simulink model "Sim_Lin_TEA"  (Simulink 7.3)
settings: Solver=ode113  StartTime=0.0  StopTime=100000  RelTol=1e-3
InitFcn:
  | start3
StopFcn:
  | Pl3
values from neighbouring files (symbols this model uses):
  Kpqr = lqr(sys,Q0,R0)    [des.m]
  r2d = 180/pi    (= 57.2957795131)    [start.m]    (also in start1.m; start2.m; start3.m)
  wo = 0.0011    [start.m]    (also in start1.m; start2.m; start3.m)
undefined symbols (not defined in the file or in its folder): Linear2_LVLH

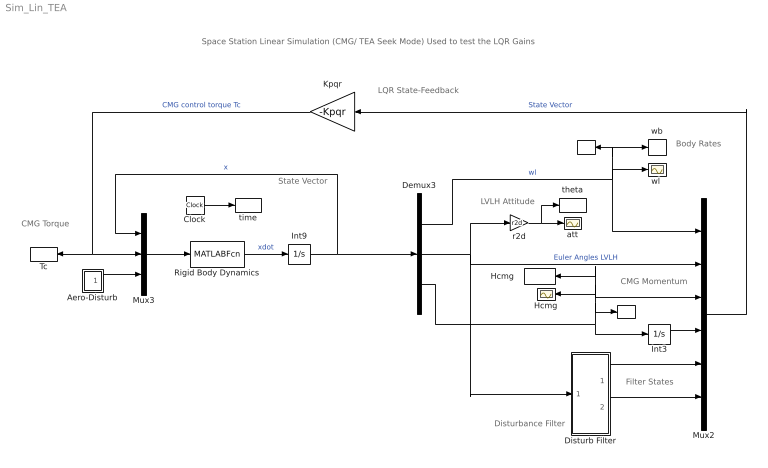
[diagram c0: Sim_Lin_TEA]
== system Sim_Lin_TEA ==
  note: Space Station Linear Simulation (CMG/ TEA Seek Mode) Used to test the LQR Gains
  note: State Vector
  note: LQR State-Feedback
  note: Body Rates
  note: CMG Momentum
  note: LVLH Attitude
  note: Filter States
  note: Disturbance Filter
  note: CMG Torque
  " " : ToWorkspace  VariableName=wl  SampleTime=-1  SaveFormat=Array
  "  " : ToWorkspace  VariableName=Hsys  SampleTime=-1  SaveFormat=Array
  Aero-Disturb : Subsystem
  Clock : Clock
  Demux3 : Demux  Outputs=[3,3,3]
  Disturb Filter : Subsystem
  Hcmg : Scope
  "Hcmg  " : ToWorkspace  VariableName=Hcmg  SampleTime=-1  SaveFormat=Array
  Int3 : Integrator
  Int9 : Integrator
  Kpqr : Gain  Gain=-Kpqr  Multiplication=Matrix(K*u)  ParameterDataType=sfix(16)  ParameterScaling=2^0  OutDataType=sfix(16)  OutScaling=2^0
  Mux2 : Mux  Inputs=[3, 3, 3, 3, 1, 1]
  Mux3 : Mux  Inputs=[9, 3, 3]
  Rigid Body Dynamics : MATLABFcn  MATLABFcn=Linear2_LVLH( u(1:9), u(10:12), u(13:15) )  OutputDimensions=9
  Tc : ToWorkspace  VariableName=Tcmg  SampleTime=-1  SaveFormat=Array
  att : Scope
  r2d : Gain  Gain=r2d  ParameterDataType=sfix(16)  ParameterScaling=2^0  OutDataType=sfix(16)  OutScaling=2^0
  theta : ToWorkspace  VariableName=theta  SampleTime=-1  SaveFormat=Array
  time : ToWorkspace  VariableName=time  SampleTime=-1  SaveFormat=Array
  wb : ToWorkspace  VariableName=wb  SampleTime=-1  SaveFormat=Array
  "wl " : Scope
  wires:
  Int3/1 -> Mux2/4
  Demux3/3 -> Int3/1, Hcmg/1, "Hcmg  "/1, Mux2/3, "  "/1
  Demux3/2 -> r2d/1, Mux2/2, Disturb Filter/1(the)  "Euler Angles LVLH"
  Kpqr/1 -> Tc/1, Mux3/2  "CMG control torque Tc"
  Int9/1 -> Demux3/1, Mux3/1  "x"
  Rigid Body Dynamics/1 -> Int9/1  "xdot"
  Demux3/1 -> "wl "/1, Mux2/1, wb/1, " "/1  "wl"
  Aero-Disturb/1(Td) -> Mux3/3
  r2d/1 -> att/1, theta/1
  Mux2/1 -> Kpqr/1  "State Vector"
  Clock/1 -> time/1
  Mux3/1 -> Rigid Body Dynamics/1
  Disturb Filter/1(a1) -> Mux2/5
  Disturb Filter/2(a2) -> Mux2/6

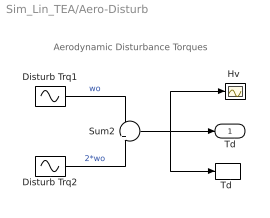
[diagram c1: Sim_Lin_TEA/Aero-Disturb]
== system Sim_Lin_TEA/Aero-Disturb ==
  note: Aerodynamic Disturbance Torques
  Disturb Trq1 : Sin  Amplitude=[1, 3, 1]  Bias="[1  8  1]"  Frequency=[wo, wo, wo]  Phase=0  Samples=10  SampleTime=0
  Disturb Trq2 : Sin  Amplitude=[1, 1, 1]*0.5  Bias=0  Frequency=[wo, wo, wo]*2  Phase=0  Samples=10  SampleTime=0
  "Hv " : Scope
  Sum2 : Sum  Inputs=+|+  OutDataType=sfix(16)  OutScaling=2^0
  "Td " : ToWorkspace  VariableName=Td  SampleTime=-1  SaveFormat=Array
  Td : Outport  OutDataType=sfix(16)  OutScaling=2^0
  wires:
  Disturb Trq2/1 -> Sum2/2  "2*wo"
  Sum2/1 -> "Td "/1, Td/1, "Hv "/1
  Disturb Trq1/1 -> Sum2/1  "wo"

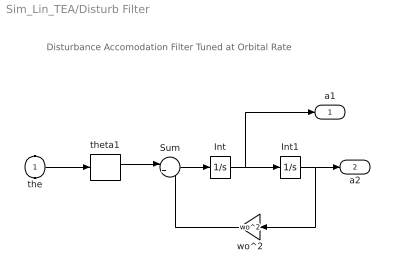
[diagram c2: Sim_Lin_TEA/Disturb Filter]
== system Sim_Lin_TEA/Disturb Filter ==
  note: Disturbance Accomodation Filter Tuned at Orbital Rate
  the : Inport  OutDataType=sfix(16)  OutScaling=2^0
  Int : Integrator
  Int1 : Integrator
  Sum : Sum  Inputs=|+-  OutDataType=sfix(16)  OutScaling=2^0
  theta1 : Selector  InputPortWidth=3  IndexOptions=Index vector (dialog)  Indices=[2]  OutputSizes=1
  wo^2 : Gain  Gain=wo^2  ParameterDataType=sfix(16)  ParameterScaling=2^0  OutDataType=sfix(16)  OutScaling=2^0
  a1 : Outport  OutDataType=sfix(16)  OutScaling=2^0
  a2 : Outport  Port=2  OutDataType=sfix(16)  OutScaling=2^0
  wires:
  Int/1 -> Int1/1, a1/1
  Sum/1 -> Int/1
  Int1/1 -> wo^2/1, a2/1
  wo^2/1 -> Sum/2
  theta1/1 -> Sum/1
  the/1 -> theta1/1
